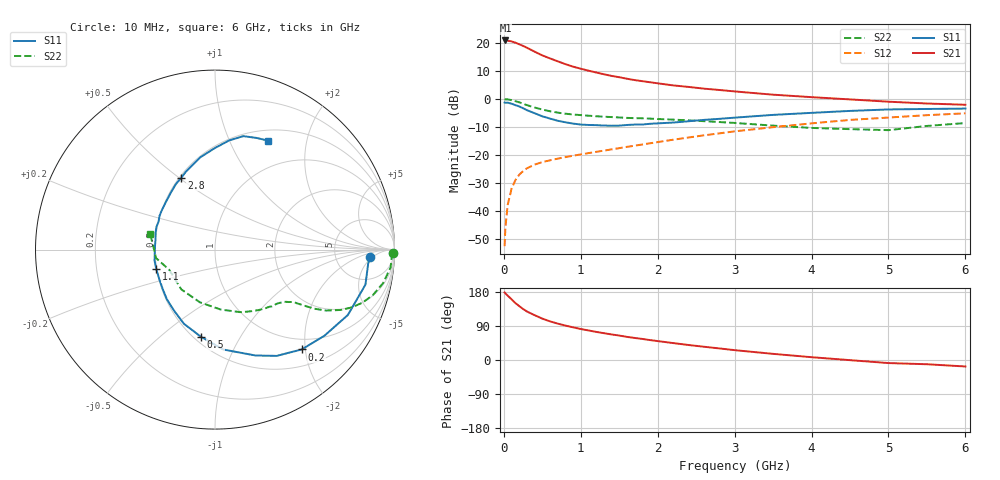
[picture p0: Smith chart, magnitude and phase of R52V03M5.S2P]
! SIEMENS Small Signal Semiconductors
! BFR183
! Si NPN RF Bipolar Junction Transistor in SOT23
! VCE = 2 V  IC = 3.5 mA
! Common Emitter S-Parameters:  May  1996
# GHz  S  MA  R  50
!  f  S11  S21  S12  S22
! GHz  MAG  ANG  MAG  ANG  MAG  ANG  MAG  ANG
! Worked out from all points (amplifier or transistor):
!   36 points, 10 MHz to 6 GHz, reference 50 ohm
!   highest |S21| = 20.8 dB at 20 MHz (marker M1)
!   |S21| within 3 dB of that: start of sweep to 329.3 MHz
!   unconditionally stable (mu >= 1): 1.184 GHz to 2.736 GHz
!   at 250 MHz: K = 0.33, MSG = 22.3 dB, |S12| = -25.7 dB
!   at 1.4 GHz: K = 1.06, MAG = 11.6 dB, |S12| = -17.9 dB
!   at 6 GHz: K = 0.90, MSG = 1.5 dB, |S12| = -5.1 dB
!   S11 on the Smith chart (normalised r, x): 10 MHz: 13, -4; 200 MHz: 0.79, -1.93; 500 MHz: 0.54, -0.69; 1.1 GHz: 0.50, -0.12; 2.8 GHz: 0.51, +0.51; 6 GHz: 0.63, +1.40
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0.01  0.8661 -2.6  10.96 178.2  0.0024 88.2  0.9934 -1.1
0.02  0.8569 -5.3  11.01 175.8  0.0051 90.3  0.9855 -2.3
0.05  0.8607 -13.1  10.88 169.9  0.013 83.0  0.9833 -5.8
0.1  0.8251 -26.2  10.59 160.2  0.0253 77.0  0.9557 -11.2
0.15  0.7762 -38.1  10.06 150.2  0.0359 69.9  0.9153 -16.1
0.2  0.7371 -49.0  9.422 142.3  0.0449 65.8  0.8719 -19.9
0.25  0.6845 -59.9  8.812 134.6  0.0519 61.6  0.8238 -23.1
0.3  0.6315 -69.1  8.171 128.0  0.0584 58.4  0.7782 -25.6
0.4  0.5585 -85.3  6.955 118.2  0.068 54.0  0.7051 -28.8
0.5  0.4917 -99.2  5.965 109.2  0.0751 51.1  0.6485 -30.6
0.6  0.448 -112.8  5.277 102.0  0.0811 50.3  0.6048 -31.7
0.7  0.4097 -123.8  4.682 96.0  0.0866 50.2  0.5722 -32.5
0.9  0.3646 -143.1  3.763 86.2  0.0978 50.5  0.5297 -33.6
1.1  0.3448 -161.7  3.193 78.0  0.1088 51.6  0.5043 -35.4
1.3  0.3364 -176.4  2.756 70.8  0.1205 52.9  0.4837 -37.0
1.6  0.3448 163.7  2.292 61.0  0.1406 54.5  0.461 -40.5
2.2  0.3805 136.2  1.746 44.7  0.1882 55.0  0.4294 -49.8
2.8  0.4429 115.0  1.447 30.6  0.2443 52.3  0.3889 -62.8
3.5  0.5212 98.9  1.193 16.2  0.3147 45.7  0.3354 -84.6
4.5  0.6133 82.6  0.983 -0.4  0.4241 33.9  0.2905 -130.3
5.5  0.6641 69.5  0.831 -11.2  0.5151 20.6  0.3313 -171.7
6  0.6749 64.0  0.789 -17.1  0.5558 12.2  0.3728 166.1
